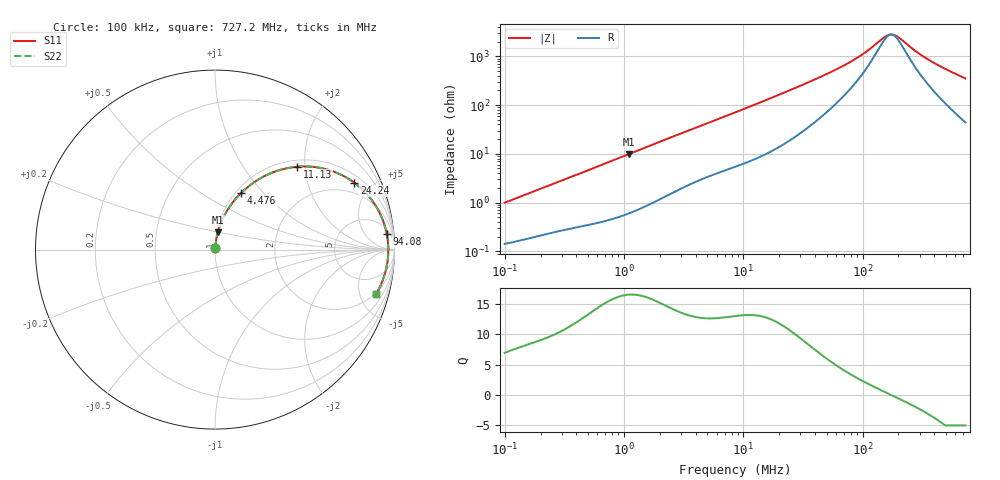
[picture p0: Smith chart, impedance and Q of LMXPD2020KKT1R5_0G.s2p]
! LMXPD2020KKT1R5_0G  S-PARAMETER MODEL  ( General Type )
! Model Generated by TAIYO YUDEN Corporation (https://www.yuden.co.jp/en/)
! Version 1.0
! TAIYO YUDEN Control No. 191023NI43SB-FBB
! Copyright(c) 2019 TAIYO YUDEN CO.,LTD. All Rights Reserved.
! Product Description (link to TY-COMPAS)
! https://ds.yuden.co.jp/TYCOMPAS/or/detail?pn=LMXPD2020KKT1R5M0G&u=M
! Products Name : Inductors
! Characteristics :
!  Inductance : 1.5 uH , SRF(min) : -Hz , DC Resistance(max) : 0.12 Ohm
!  Rated Current : Saturation :1350 mA , Temp Rise : 1450 mA (40 degC)
!  Case Size : 2.0 x 2.0 / 0.079 x 0.079 [mm/inch] , Thickness : 1 / 0.039 [mm/inch]
!  (Conditions: Temperature = 25 degC , DC Bias Current/Voltage = 0A / 0V)
! External Node Assignments :
!  1  o---GGG---o  2
! GND o---------o GND
! Frequency Range : 0.1MHz  -  727.209926MHz  [ 402 STEP ]
# MHz S RI R 50
! Freq[MHz].  S11 Real  S11 Imag  S21 Real  S21 Imag  S12 Real  S12 Imag  S22 Real  S22 Imag
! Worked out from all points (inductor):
!   401 points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, 100 kHz to 727.2 MHz, reference 50 ohm
!   read as one part in series: L = 1.55 uH near 104.5 kHz
!   highest Q = 16.5 at 1.103 MHz (marker M1), where L = 1.43 uH
!   self-resonance near 174 MHz
!   S11 on the Smith chart (normalised r, x): 100 kHz: 1.00, +0.02; 4.476 MHz: 1.06, +0.76; 11.13 MHz: 1.14, +1.82; 24.24 MHz: 1.37, +3.95; 94.08 MHz: 8, +19; 727.2 MHz: 1.88, -6.98
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0.1  0.00151 0.0098  0.9985 -0.0098  0.9985 -0.0098  0.00151 0.0098
0.443433  0.00487 0.0404  0.9951 -0.0404  0.9951 -0.0404  0.00487 0.0404
1.103184  0.0155 0.0969  0.9845 -0.0969  0.9845 -0.0969  0.0155 0.0969
1.966328  0.0396 0.165  0.9604 -0.165  0.9604 -0.165  0.0396 0.165
3.067178  0.0818 0.2394  0.9182 -0.2394  0.9182 -0.2394  0.0818 0.2394
4.475686  0.1453 0.3152  0.8547 -0.3152  0.8547 -0.3152  0.1453 0.3152
6.247004  0.2315 0.3842  0.7685 -0.3842  0.7685 -0.3842  0.2315 0.3842
8.719349  0.3511 0.4404  0.6489 -0.4404  0.6489 -0.4404  0.3511 0.4404
11.13473  0.4567 0.4616  0.5433 -0.4616  0.5433 -0.4616  0.4567 0.4616
15.89081  0.6174 0.4482  0.3826 -0.4482  0.3826 -0.4482  0.6174 0.4482
24.24236  0.7769 0.3723  0.2231 -0.3723  0.2231 -0.3723  0.7769 0.3723
37.81446  0.8814 0.2654  0.1186 -0.2654  0.1186 -0.2654  0.8814 0.2654
63.05265  0.9385 0.1552  0.0615 -0.1552  0.0615 -0.1552  0.9385 0.1552
94.07583  0.9572 0.0865  0.0428 -0.0865  0.0428 -0.0865  0.9572 0.0865
150.0428  0.9651 0.0198  0.0349 -0.0198  0.0349 -0.0198  0.9651 0.0198
167.6818  0.9655 0.00492  0.0345 -0.00492  0.0345 -0.00492  0.9655 0.00492
179.2455  0.9656 -0.00398  0.0344 0.00398  0.0344 0.00398  0.9656 -0.00398
195.9138  0.9654 -0.0159  0.0346 0.0159  0.0346 0.0159  0.9654 -0.0159
285.8811  0.9608 -0.0687  0.0392 0.0687  0.0392 0.0687  0.9608 -0.0687
390.2506  0.951 -0.1182  0.049 0.1182  0.049 0.1182  0.951 -0.1182
544.6981  0.9306 -0.1809  0.0694 0.1809  0.0694 0.1809  0.9306 -0.1809
727.2099  0.899 -0.2449  0.101 0.2449  0.101 0.2449  0.899 -0.2449
